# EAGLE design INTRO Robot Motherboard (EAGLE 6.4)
Schematic of the Motherboard from the INTRO Robot
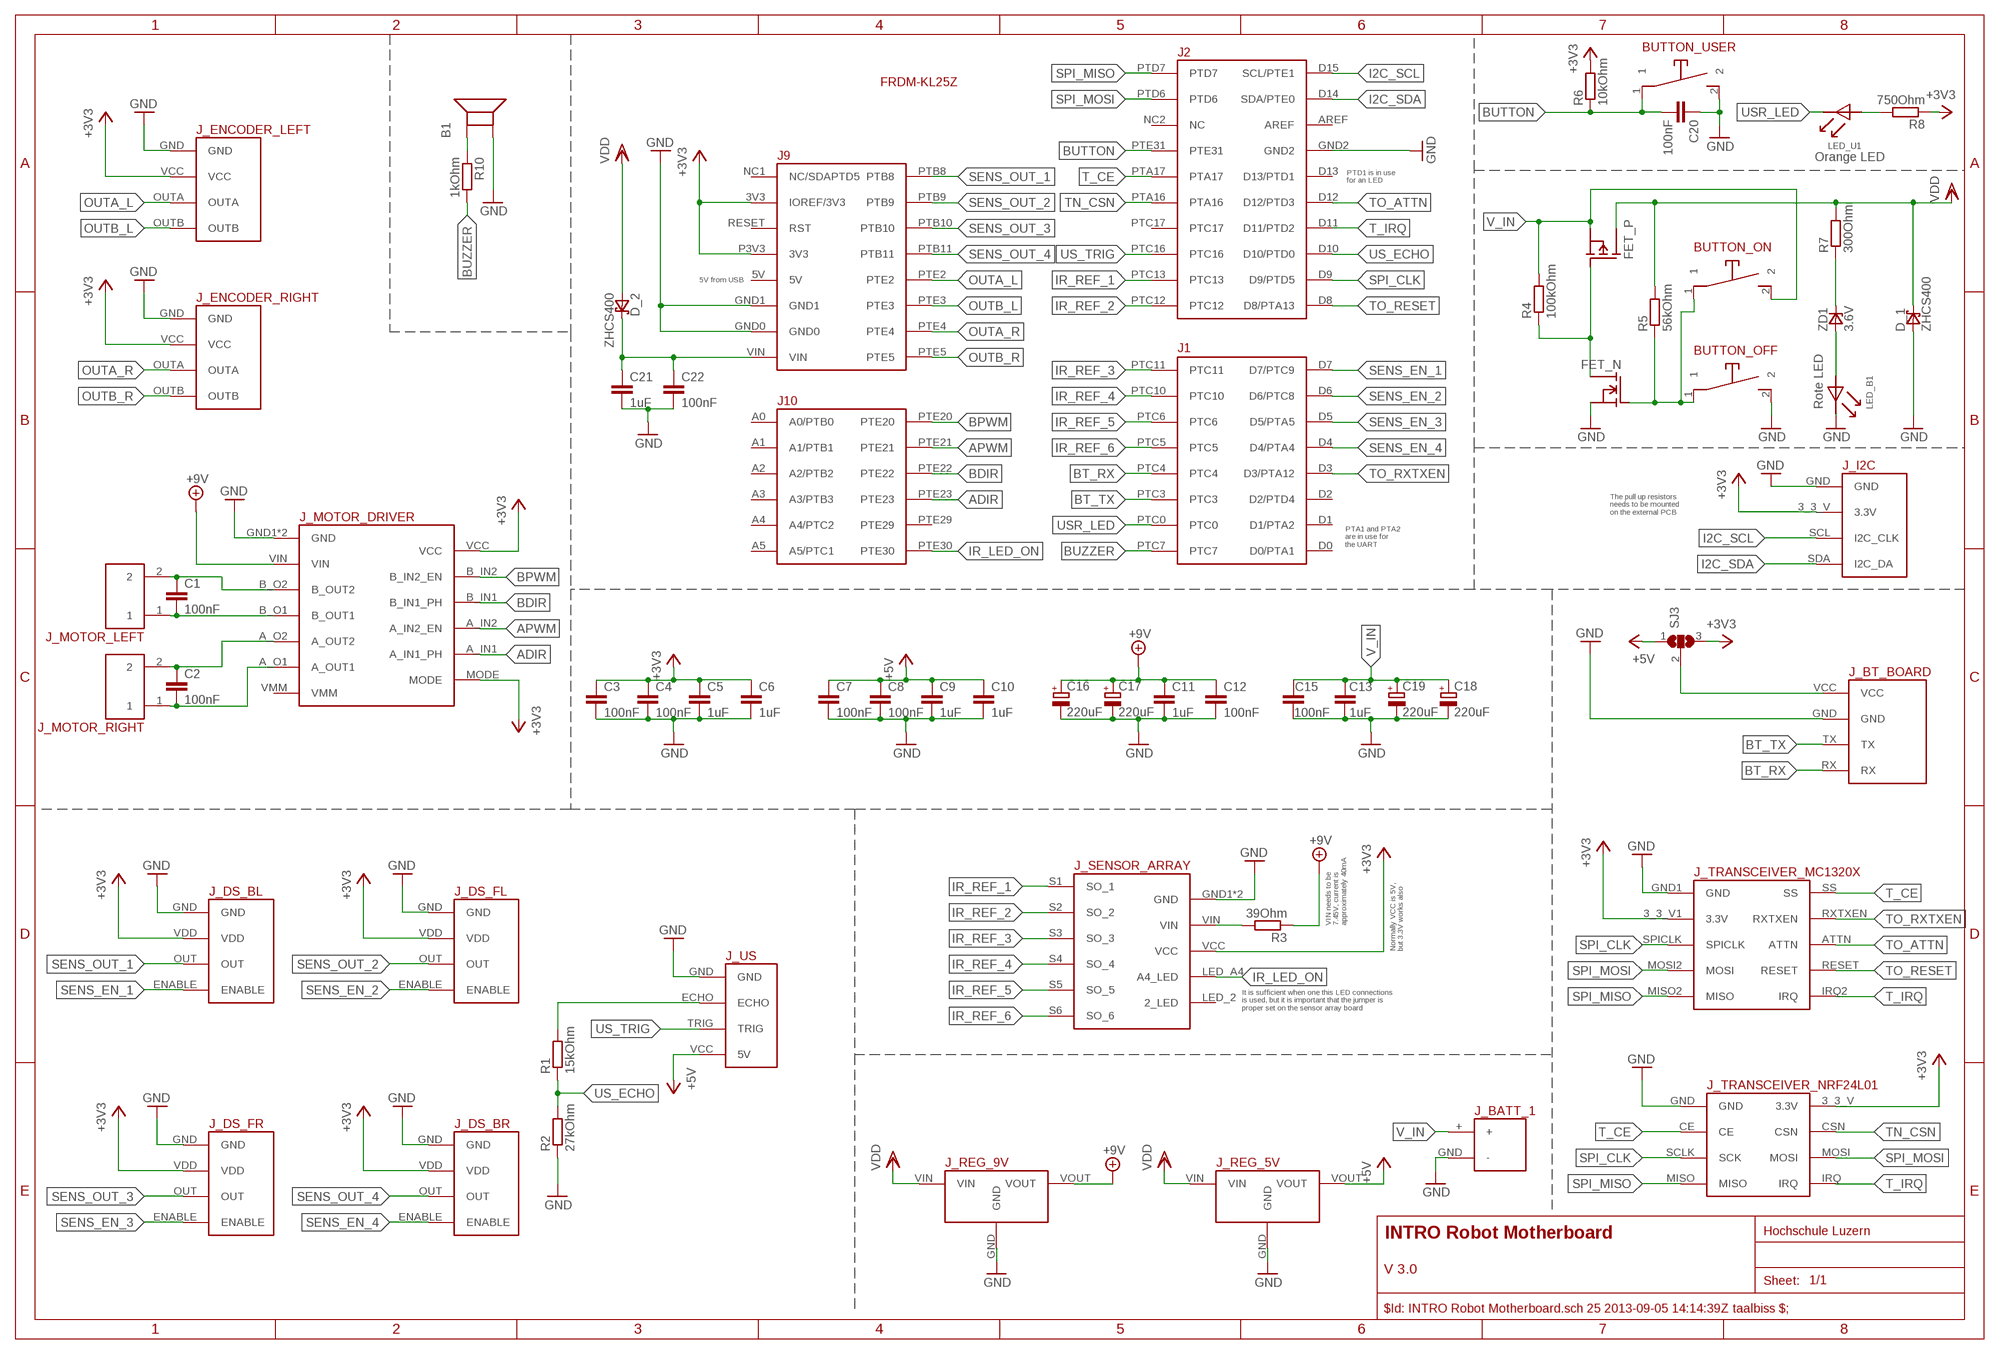
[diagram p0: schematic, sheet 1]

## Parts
B1  BUZZER  [BUZZER]
BUTTON_OFF  MINI_PUSHBUTTON  [MINI_PUSHBUTTON_FOOTPRINT]
BUTTON_ON  MINI_PUSHBUTTON  [MINI_PUSHBUTTON_FOOTPRINT]
BUTTON_USER  MINI_PUSHBUTTON  [MINI_PUSHBUTTON_FOOTPRINT]
C1  100nF  C-EUC0805  [C0805]
C2  100nF  C-EUC0805  [C0805]
C3  100nF  C-EUC0805  [C0805]
C4  100nF  C-EUC0805  [C0805]
C5  1uF  C-EUC0805  [C0805]
C6  1uF  C-EUC0805  [C0805]
C7  100nF  C-EUC0805  [C0805]
C8  100nF  C-EUC0805  [C0805]
C9  1uF  C-EUC0805  [C0805]
C10  1uF  C-EUC0805  [C0805]
C11  1uF  C-EUC0805  [C0805]
C12  100nF  C-EUC0805  [C0805]
C13  1uF  C-EUC0805  [C0805]
C15  100nF  C-EUC0805  [C0805]
C16  220uF  CPOL-EU153CLV-0605  [153CLV-0605]
C17  220uF  CPOL-EU153CLV-0605  [153CLV-0605]
C18  220uF  CPOL-EU153CLV-0605  [153CLV-0605]
C19  220uF  CPOL-EU153CLV-0605  [153CLV-0605]
C20  100nF  C-EUC0805  [C0805]
C21  1uF  C-EUC0805  [C0805]
C22  100nF  C-EUC0805  [C0805]
D_1  ZHCS400  SCHOTTKY_ZHCS400  [SOD-323]
D_2  ZHCS400  SCHOTTKY_ZHCS400  [SOD-323]
FET_N  NFET_SOT23  [SOT-23]
FET_P  PFET_SOT23  [SOT-23]
FRDM1  FRDM-KL25ZARDUINO  [FRDM-KL25Z]
J_BATT_1  BATTERY_CONNECTION  [BATTERY_CONNECTION_FOOTPRINT]
J_BT_BOARD  BLUETOOTH_BOARD  [BT_BOARD_FOOTPRINT]
J_DS_BL  POLOLU_DIST_PROX_SENS  [POLOLU_DIST_PROX_SENS_FOOTPRINT]
J_DS_BR  POLOLU_DIST_PROX_SENS  [POLOLU_DIST_PROX_SENS_FOOTPRINT]
J_DS_FL  POLOLU_DIST_PROX_SENS  [POLOLU_DIST_PROX_SENS_FOOTPRINT]
J_DS_FR  POLOLU_DIST_PROX_SENS  [POLOLU_DIST_PROX_SENS_FOOTPRINT]
J_ENCODER_LEFT  ENCODER  [ENCODER_FOOTPRINT]
J_ENCODER_RIGHT  ENCODER  [ENCODER_FOOTPRINT]
J_I2C  I2C_HEADER  [I2C_HEADER_FOOTPRINT]
J_MOTOR_DRIVER  MOTOR_DRIVER  [MOTOR_DRIVER_FOOTPRINT]
J_MOTOR_LEFT  MOTOR_CONNECTOR  [MOTOR_CONNECTOR_FOOTPRINT]
J_MOTOR_RIGHT  MOTOR_CONNECTOR  [MOTOR_CONNECTOR_FOOTPRINT]
J_REG_5V  5V_VOLTAGE_REGULATOR  [5V_VOLTAGE_REGULATOR]
J_REG_9V  9V_VOLTAGE_REGULATOR  [9V_VOLTAGE_REGULATOR]
J_SENSOR_ARRAY  REFLECTANCE_SENSOR_ARRAY  [REFLECTANCE_SENSOR_ARRAY_FOOTPRINT]
J_TRANSCEIVER  MC1320X_AND_NRF24L01  [MC1320X_AND_NRF24L01_FOOTPRINT]
J_US  HC-SR04  [HC-SR04_FOOTPRINT]
LED_B1  LED_PLCC-2  [PLCC-2]
LED_U1  LED_PLCC-2  [PLCC-2]
R1  15kOhm  R-EU_R0805  [R0805]
R2  27kOhm  R-EU_R0805  [R0805]
R3  39Ohm  R-EU_R0805  [R0805]
R4  100kOhm  R-EU_R0805  [R0805]
R5  56kOhm  R-EU_R0805  [R0805]
R6  10kOhm  R-EU_R0805  [R0805]
R7  300Ohm  R-EU_R0805  [R0805]
R8  750Ohm  R-EU_R0805  [R0805]
R10  1kOhm  R-EU_R0805  [R0805]
SJ3  SJ2W  [SJ_2]
ZD1  3.6V  ZDIODE_SOD323  [SOD-323]

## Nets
+3V3: C3.1 C4.1 C5.1 C6.1 FRDM1.3V3(IOREF/3V3) FRDM1.P3V3(3V3) J_DS_BL.VDD J_DS_BR.VDD J_DS_FL.VDD J_DS_FR.VDD J_ENCODER_LEFT.VCC J_ENCODER_RIGHT.VCC J_I2C.3_3_V(3.3V) J_MOTOR_DRIVER.MODE J_MOTOR_DRIVER.VCC J_SENSOR_ARRAY.VCC J_TRANSCEIVER.3_3_V1(_MC1320X:3.3V) J_TRANSCEIVER.3_3_V(_NRF24L01:3.3V) R6.2 R8.1 SJ3.3
+5V: C7.1 C8.1 C9.1 C10.1 J_REG_5V.VOUT J_US.VCC(5V) SJ3.1
+9V: C11.1 C12.1 C16.+ C17.+ J_MOTOR_DRIVER.VIN J_REG_9V.VOUT R3.1
ADIR: FRDM1.PTE23 J_MOTOR_DRIVER.A_IN1(A_IN1_PH)
APWM: FRDM1.PTE21 J_MOTOR_DRIVER.A_IN2(A_IN2_EN)
BDIR: FRDM1.PTE22 J_MOTOR_DRIVER.B_IN1(B_IN1_PH)
BPWM: FRDM1.PTE20 J_MOTOR_DRIVER.B_IN2(B_IN2_EN)
BT_RX: FRDM1.PTC4 J_BT_BOARD.RX
BT_TX: FRDM1.PTC3 J_BT_BOARD.TX
BUTTON: BUTTON_USER.1 C20.2 FRDM1.PTE31 R6.1
BUZZER: FRDM1.PTC7 R10.2
GND: B1.2 BUTTON_OFF.2 BUTTON_USER.2 C3.2 C4.2 C5.2 C6.2 C7.2 C8.2 C9.2 C10.2 C11.2 C12.2 C13.1 C15.1 C16.- C17.- C18.- C19.- C20.1 C21.2 C22.2 D_1.1(A) FET_N.2(S) FRDM1.GND0 FRDM1.GND1 FRDM1.GND2 J_BATT_1.GND(-) J_BT_BOARD.GND J_DS_BL.GND J_DS_BR.GND J_DS_FL.GND J_DS_FR.GND J_ENCODER_LEFT.GND J_ENCODER_RIGHT.GND J_I2C.GND J_MOTOR_DRIVER.GND1(GND) J_MOTOR_DRIVER.GND2(GND) J_REG_5V.GND J_REG_9V.GND J_SENSOR_ARRAY.GND1(GND) J_SENSOR_ARRAY.GND2(GND) J_TRANSCEIVER.GND1(_MC1320X:GND) J_TRANSCEIVER.GND(_NRF24L01:GND) J_US.GND LED_B1.K R2.1
I2C_SCL: FRDM1.D15(SCL/PTE1) J_I2C.SCL(I2C_CLK)
I2C_SDA: FRDM1.D14(SDA/PTE0) J_I2C.SDA(I2C_DA)
IR_LED_ON: FRDM1.PTE30 J_SENSOR_ARRAY.LED_A4(A4_LED)
IR_REF_1: FRDM1.PTC13 J_SENSOR_ARRAY.S1(SO_1)
IR_REF_2: FRDM1.PTC12 J_SENSOR_ARRAY.S2(SO_2)
IR_REF_3: FRDM1.PTC11 J_SENSOR_ARRAY.S3(SO_3)
IR_REF_4: FRDM1.PTC10 J_SENSOR_ARRAY.S4(SO_4)
IR_REF_5: FRDM1.PTC6 J_SENSOR_ARRAY.S5(SO_5)
IR_REF_6: FRDM1.PTC5 J_SENSOR_ARRAY.S6(SO_6)
N$1: C1.1 J_MOTOR_DRIVER.B_O2(B_OUT2) J_MOTOR_LEFT.2
N$2: J_US.ECHO R1.2
N$3: C2.1 J_MOTOR_DRIVER.A_O2(A_OUT2) J_MOTOR_RIGHT.2
N$4: C1.2 J_MOTOR_DRIVER.B_O1(B_OUT1) J_MOTOR_LEFT.1
N$5: C2.2 J_MOTOR_DRIVER.A_O1(A_OUT1) J_MOTOR_RIGHT.1
N$6: J_SENSOR_ARRAY.VIN R3.2
N$7: C21.1 C22.1 D_2.2(C) FRDM1.VIN
N$8: FET_N.1(D) FET_P.3(G) R4.1
N$9: J_BT_BOARD.VCC SJ3.2
N$10: LED_B1.A ZD1.2(A)
N$11: BUTTON_OFF.1 BUTTON_ON.1 FET_N.3(G) R5.1
N$12: R7.1 ZD1.1(C)
N$15: LED_U1.A R8.2
N$16: B1.1 R10.1
OUTA_L: FRDM1.PTE2 J_ENCODER_LEFT.OUTA
OUTA_R: FRDM1.PTE4 J_ENCODER_RIGHT.OUTA
OUTB_L: FRDM1.PTE3 J_ENCODER_LEFT.OUTB
OUTB_R: FRDM1.PTE5 J_ENCODER_RIGHT.OUTB
SENS_EN_1: FRDM1.D7(D7/PTC9) J_DS_BL.ENABLE
SENS_EN_2: FRDM1.D6(D6/PTC8) J_DS_FL.ENABLE
SENS_EN_3: FRDM1.D5(D5/PTA5) J_DS_FR.ENABLE
SENS_EN_4: FRDM1.D4(D4/PTA4) J_DS_BR.ENABLE
SENS_OUT_1: FRDM1.PTB8 J_DS_BL.OUT
SENS_OUT_2: FRDM1.PTB9 J_DS_FL.OUT
SENS_OUT_3: FRDM1.PTB10 J_DS_FR.OUT
SENS_OUT_4: FRDM1.PTB11 J_DS_BR.OUT
SPI_CLK: FRDM1.D9(D9/PTD5) J_TRANSCEIVER.SCLK(_NRF24L01:SCK) J_TRANSCEIVER.SPICLK(_MC1320X:SPICLK)
SPI_MISO: FRDM1.PTD7 J_TRANSCEIVER.MISO2(_MC1320X:MISO) J_TRANSCEIVER.MISO(_NRF24L01:MISO)
SPI_MOSI: FRDM1.PTD6 J_TRANSCEIVER.MOSI2(_MC1320X:MOSI) J_TRANSCEIVER.MOSI(_NRF24L01:MOSI)
T_CE: FRDM1.PTA17 J_TRANSCEIVER.CE(_NRF24L01:CE) J_TRANSCEIVER.SS(_MC1320X:SS)
T_IRQ: FRDM1.D11(D11/PTD2) J_TRANSCEIVER.IRQ2(_MC1320X:IRQ) J_TRANSCEIVER.IRQ(_NRF24L01:IRQ)
TN_CSN: FRDM1.PTA16 J_TRANSCEIVER.CSN(_NRF24L01:CSN)
TO_ATTN: FRDM1.D12(D12/PTD3) J_TRANSCEIVER.ATTN(_MC1320X:ATTN)
TO_RESET: FRDM1.D8(D8/PTA13) J_TRANSCEIVER.RESET(_MC1320X:RESET)
TO_RXTXEN: FRDM1.D3(D3/PTA12) J_TRANSCEIVER.RXTXEN(_MC1320X:RXTXEN)
US_ECHO: FRDM1.D10(D10/PTD0) R1.1 R2.2
US_TRIG: FRDM1.PTC16 J_US.TRIG
USR_LED: FRDM1.PTC0 LED_U1.K
V_IN: BUTTON_ON.2 C13.2 C15.2 C18.+ C19.+ FET_P.2(S) J_BATT_1.+ R4.2
VDD: D_1.2(C) D_2.1(A) FET_P.1(D) J_REG_5V.VIN J_REG_9V.VIN R5.2 R7.2
Unconnected: FRDM1.5V FRDM1.A0(A0/PTB0) FRDM1.A1(A1/PTB1) FRDM1.A2(A2/PTB2) FRDM1.A3(A3/PTB3) FRDM1.A4(A4/PTC2) FRDM1.A5(A5/PTC1) FRDM1.AREF FRDM1.D0(D0/PTA1) FRDM1.D1(D1/PTA2) FRDM1.D2(D2/PTD4) FRDM1.D13(D13/PTD1) FRDM1.NC1(NC/SDAPTD5) FRDM1.NC2(NC) FRDM1.PTC17 FRDM1.PTE29 FRDM1.RESET(RST) J_MOTOR_DRIVER.VMM J_SENSOR_ARRAY.LED_2(2_LED)

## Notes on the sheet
- Orange LED
- PTD1 is in use
  for an LED
- 5V from USB
- Rote LED
- The pull up resistors 
  needs to be mounted 
  on the external PCB
- PTA1 and PTA2
  are in use for 
  the UART
- VIN needs to be 
  7.45V, current is 
  approximately 40mA
- Normally VCC is 5V, 
  but 3.3V works also
- It is sufficient when one this LED connections 
  is used, but it is important that the jumper is 
  proper set on the sensor array board
- V 3.0
- $Id: INTRO Robot Motherboard.sch 25 2013-09-05 14:14:39Z taalbiss $;

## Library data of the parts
B1 = INTRO_Robot_Miscellaneous:BUZZER
BUTTON_OFF BUTTON_ON BUTTON_USER = Pololu Button:MINI_PUSHBUTTON: Mini Pushbutton Switch, 2-Pin, SPST, 50mA
C1-C13 C15 C20-C22 = rcl:C-EU: CAPACITOR, European symbol
C16-C19 = rcl:CPOL-EU: POLARIZED CAPACITOR, European symbol
D_1 D_2 = INTRO_Robot_Miscellaneous:SCHOTTKY_ZHCS400
FET_N = INTRO_Robot_Miscellaneous:NFET_SOT23
FET_P = INTRO_Robot_Miscellaneous:PFET_SOT23
FRDM1 = Freedom:FRDM-KL25Z: For creating FRDM-KL25Z shields
J_BATT_1 = Zumo Robot Battery Connection:BATTERY_CONNECTION: Battery Connection for the Zuma Robot
J_BT_BOARD = Bluetooth HC-05:BLUETOOTH_BOARD: Bluetooth Board V1.05
J_DS_BL J_DS_BR J_DS_FL J_DS_FR = Pololu Digital Distance and Proximity Sensors:POLOLU_DIST_PROX_SENS: Pololu Digital Distance and Proximity Sensors; Pololu Items Nr. 1134; 1132; 2460; 2461
J_ENCODER_LEFT J_ENCODER_RIGHT = Pololu Encoder and Motor Driver:ENCODER: Encoder for Pololu Wheel 42x19mm
J_I2C = I2C_Header:I2C_HEADER
J_MOTOR_DRIVER = Pololu Encoder and Motor Driver:MOTOR_DRIVER: DRV8835 Dual Motor Driver Carrier
J_MOTOR_LEFT J_MOTOR_RIGHT = Pololu Encoder and Motor Driver:MOTOR_CONNECTOR: Connector for a Motor
J_REG_5V = Pololu Voltage Regulators:5V_VOLTAGE_REGULATOR: Polulu 5V Step-Up/Step-Down Voltage REgulator S7V7F5
J_REG_9V = Pololu Voltage Regulators:9V_VOLTAGE_REGULATOR: Polulu 9V Step-Up Voltage Regulator U3V12F9
J_SENSOR_ARRAY = Pololu Zumo Reflectance Sensor Array:REFLECTANCE_SENSOR_ARRAY: Zumo Reflectance Sensor Array Item #1419
J_TRANSCEIVER = Nordic Semiconductors 2.4GHz Transceiver:MC1320X_AND_NRF24L01: With this Device, it is possible to use the NRF24L01 or the MC1320x 802.15.4 transceiver
J_US = Ultrasonic Sensor HC-SR04:HC-SR04: Ultrasonic Sensor HC-SR04
LED_B1 LED_U1 = INTRO_Robot_Miscellaneous:LED_PLCC-2
R1-R8 R10 = rcl:R-EU_: RESISTOR, European symbol
SJ3 = jumper:SJ2W: SMD solder JUMPER
ZD1 = INTRO_Robot_Miscellaneous:ZDIODE_SOD323

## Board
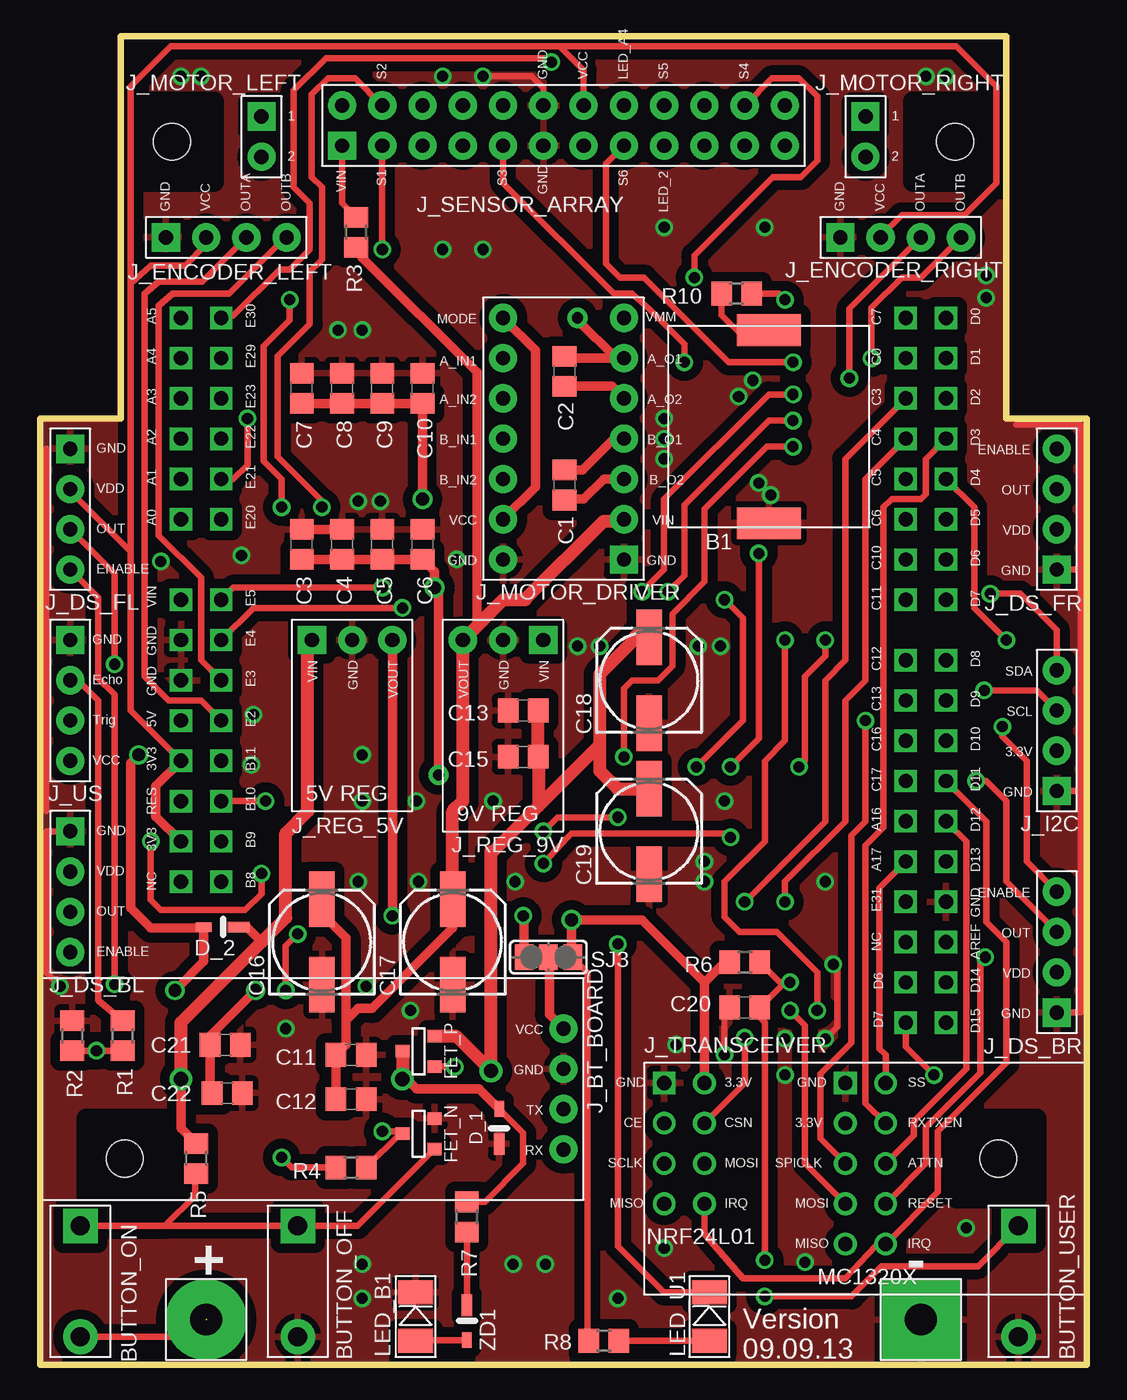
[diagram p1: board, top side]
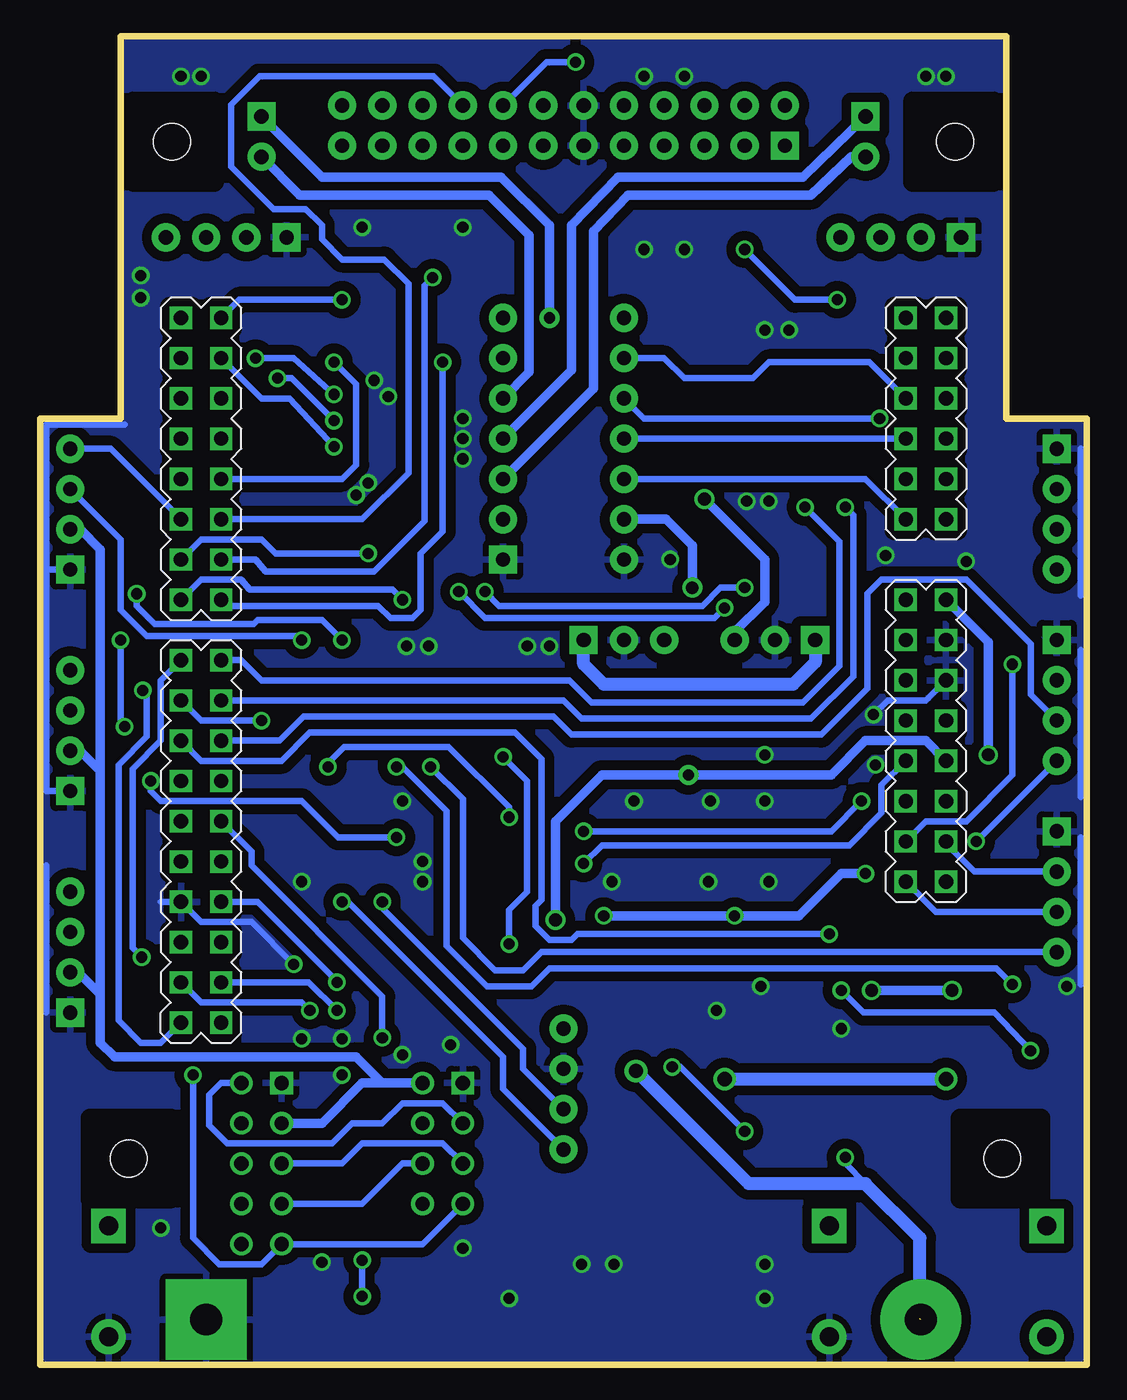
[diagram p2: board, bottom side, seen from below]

No outline drawn. Coordinates in mm, seen from the top.
Copper layers (1*16): 46 0.035mm / dielectric 1.5mm / Bottom 0.035mm
Design rules "default *": minimum track width 10mil, minimum drill 24mil, track to track 10mil, track to pad 10mil, pad to pad 20mil, via to via 20mil, smd to smd 8mil, copper to edge 40mil, drill to drill 10mil, minimum pad ring 10mil, minimum via ring 8mil, stop-mask expansion 4mil, vias tented up to drill 0mil, thermal gap 15mil
Holes 2.31 mm at 5.33,13.02 60.45,13.02 57.72,77.15 8.32,77.15
tRestrict: area 2.9,10.5 to 8,15.6; area 57.8,10.5 to 62.9,15.6; area 5.9,74.6 to 11,79.7; area 55.1,74.6 to 60.1,79.7
bRestrict: area 2.9,10.5 to 8,15.6; area 57.8,10.5 to 62.9,15.6; area 55.1,74.6 to 60.1,79.7; area 5.9,74.6 to 11,79.7
Milling: 8 lines

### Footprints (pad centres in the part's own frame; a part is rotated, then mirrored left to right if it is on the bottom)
BUZZER = smd 2.007 x 4.013: 1 -6.096,0; 2 6.096,0
MINI_PUSHBUTTON_FOOTPRINT = drill 1.2 pad 2.184 square: 1 -3.81,0 | drill 1.2 pad 2.184: 2 3.175,0
C0805 = smd 1.3 x 1.5: 1 -0.95,0; 2 0.95,0
153CLV-0605 = smd 3.5 x 1.6: + 2.7,0; - -2.7,0
SOD-323 = smd 1.397 x 0.66: 1 -1.1,0 | smd 1 x 0.6: 2 1.1,0
SOT-23 = smd 0.787 x 0.889: 1 0.025,-1.016; 2 -0.94,1.016; 3 0.991,1.016
FRDM-KL25Z = drill 0.9 square: 3V3 -22.86,-8.89; 5V -22.86,-1.27; A0 -22.86,11.43; A1 -22.86,13.97; A2 -22.86,16.51; A3 -22.86,19.05; A4 -22.86,21.59; A5 -22.86,24.13; AREF 25.4,-15.24; D0 25.4,24.13; D1 25.4,21.59; D2 25.4,19.05; D3 25.4,16.51; D4 25.4,13.97; D5 25.4,11.43; D6 25.4,8.89; D7 25.4,6.35; D8 25.4,2.54; D9 25.4,0; D10 25.4,-2.54; D11 25.4,-5.08; D12 25.4,-7.62; D13 25.4,-10.16; D14 25.4,-17.78; D15 25.4,-20.32; GND0 -22.86,3.81; GND1 -22.86,1.27; GND2 25.4,-12.7; NC1 -22.86,-11.43; NC2 22.86,-15.24; P3V3 -22.86,-3.81; PTA16 22.86,-7.62; PTA17 22.86,-10.16; PTB8 -20.32,-11.43; PTB9 -20.32,-8.89; PTB10 -20.32,-6.35; PTB11 -20.32,-3.81; PTC0 22.86,21.59; PTC3 22.86,19.05; PTC4 22.86,16.51; PTC5 22.86,13.97; PTC6 22.86,11.43; PTC7 22.86,24.13; PTC10 22.86,8.89; PTC11 22.86,6.35; PTC12 22.86,2.54; PTC13 22.86,0; PTC16 22.86,-2.54; PTC17 22.86,-5.08; PTD6 22.86,-17.78; PTD7 22.86,-20.32; PTE2 -20.32,-1.27; PTE3 -20.32,1.27; PTE4 -20.32,3.81; PTE5 -20.32,6.35; PTE20 -20.32,11.43; PTE21 -20.32,13.97; PTE22 -20.32,16.51; PTE23 -20.32,19.05; PTE29 -20.32,21.59; PTE30 -20.32,24.13; PTE31 22.86,-12.7; RESET -22.86,-6.35; VIN -22.86,6.35
BATTERY_CONNECTION_FOOTPRINT = drill 2 pad 5.08: + -22.86,0 | drill 2 pad 5.08 square: GND 22.225,0
BT_BOARD_FOOTPRINT = drill 0.9 pad 1.778: GND -16.51,-1.27; RX -16.51,3.81; TX -16.51,1.27; VCC -16.51,-3.81
POLOLU_DIST_PROX_SENS_FOOTPRINT = drill 0.9 pad 1.778: ENABLE 0,-3.81; OUT 0,-1.27; VDD 0,1.27 | drill 0.9 pad 1.778 square: GND 0,3.81
ENCODER_FOOTPRINT = drill 0.9 pad 1.778 square: GND -3.81,0 | drill 0.9 pad 1.778: OUTA 1.27,0; OUTB 3.81,0; VCC -1.27,0
I2C_HEADER_FOOTPRINT = drill 0.9 pad 1.778: 3_3_V -1.27,0; SCL 1.27,0; SDA 3.81,0 | drill 0.9 pad 1.778 square: GND -3.81,0
MOTOR_DRIVER_FOOTPRINT = drill 0.9 pad 1.778: A_IN1 3.81,-5.08; A_IN2 3.81,-2.54; A_O1 -3.81,-5.08; A_O2 -3.81,-2.54; B_IN1 3.81,0; B_IN2 3.81,2.54; B_O1 -3.81,0; B_O2 -3.81,2.54; GND2 3.81,7.62; MODE 3.81,-7.62; VCC 3.81,5.08; VIN -3.81,5.08; VMM -3.81,-7.62 | drill 0.9 pad 1.778 square: GND1 -3.81,7.62
MOTOR_CONNECTOR_FOOTPRINT = drill 0.9 pad 1.778 square: 1 0,1.27 | drill 0.9 pad 1.778: 2 0,-1.27
5V_VOLTAGE_REGULATOR = drill 0.9 pad 1.778: GND 0,-6.35; VOUT -2.54,-6.35 | drill 0.9 pad 1.778 square: VIN 2.54,-6.35
9V_VOLTAGE_REGULATOR = drill 0.9 pad 1.778: GND 0,-1.27; VOUT 2.54,-1.27 | drill 0.9 pad 1.778 square: VIN -2.54,-1.27
REFLECTANCE_SENSOR_ARRAY_FOOTPRINT = drill 0.9 pad 1.778: GND1 -1.27,0; GND2 1.27,0; LED_2 -1.27,-7.62; LED_A4 1.27,-5.08; NC$4 1.27,2.54; NC$5 -1.27,5.08; NC$6 1.27,5.08; NC$7 -1.27,7.62; NC$8 1.27,7.62; NC$12 1.27,12.7; NC$15 -1.27,-2.54; NC$17 -1.27,-10.16; NC$18 1.27,-10.16; NC$21 -1.27,-12.7; NC$23 -1.27,-15.24; NC$24 1.27,-15.24; S1 -1.27,10.16; S2 1.27,10.16; S3 -1.27,2.54; S4 1.27,-12.7; S5 1.27,-7.62; S6 -1.27,-5.08; VCC 1.27,-2.54 | drill 0.9 pad 1.778 square: VIN -1.27,12.7
MC1320X_AND_NRF24L01_FOOTPRINT = drill 0.9 pad 1.422: 3_3_V -11.43,6.35; 3_3_V1 -2.54,3.81; ATTN 0,1.27; CE -13.97,3.81; CSN -11.43,3.81; IRQ -11.43,-1.27; IRQ2 0,-3.81; MISO -13.97,-1.27; MISO2 -2.54,-3.81; MOSI -11.43,1.27; MOSI2 -2.54,-1.27; RESET 0,-1.27; RXTXEN 0,3.81; SCLK -13.97,1.27; SPICLK -2.54,1.27; SS 0,6.35 | drill 0.9 pad 1.422 square: GND -13.97,6.35; GND1 -2.54,6.35
HC-SR04_FOOTPRINT = drill 0.9 pad 1.778: ECHO 0,1.27; TRIG 0,-1.27; VCC 0,-3.81 | drill 0.9 pad 1.778 square: GND 0,3.81
PLCC-2 = smd 1.499 x 2.21: A -1.524,0; K 1.524,0
R0805 = smd 1.3 x 1.5: 1 -0.95,0; 2 0.95,0
SJ_2 = smd 1.168 x 1.6: 1 -1.524,0; 2 0,0; 3 1.524,0

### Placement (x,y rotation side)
B1  45.97,59.18 270 top
BUTTON_OFF  16.26,4.95 270 top
BUTTON_ON  2.54,4.95 270 top
BUTTON_USER  61.72,4.95 270 top
C1  33.08,55.5 90 top
C2  33.08,62.67 90 top
C3  16.51,51.75 90 top
C4  19.05,51.75 90 top
C5  21.59,51.75 90 top
C6  24.13,51.75 90 top
C7  16.51,61.59 90 top
C8  19.05,61.59 90 top
C9  21.59,61.59 90 top
C10  24.13,61.59 90 top
C11  19.62,19.56 0 top
C12  19.62,16.76 0 top
C13  30.48,41.27 0 top
C15  30.48,38.35 0 top
C16  17.78,26.67 90 top
C17  26.04,26.67 90 top
C18  38.42,43.18 90 top
C19  38.42,33.66 90 top
C20  44.45,22.54 0 top
C21  11.68,20.19 0 top
C22  11.81,17.14 0 top
D_1  28.96,15.05 90 top
D_2  11.43,27.62 180 top
FET_N  23.88,14.61 270 top
FET_P  23.88,19.81 270 top
FRDM1  31.75,41.91 0 top
J_BATT_1  33.34,2.86 0 top
J_BT_BOARD  16.51,17.4 180 top
J_DS_BL  1.91,29.84 0 top
J_DS_BR  64.14,26.04 180 top
J_DS_FL  1.91,53.98 0 top
J_DS_FR  64.14,53.98 180 top
J_ENCODER_LEFT  11.75,71.12 0 top
J_ENCODER_RIGHT  54.29,71.12 0 top
J_I2C  64.14,40.01 90 top
J_MOTOR_DRIVER  33.02,58.42 180 top
J_MOTOR_LEFT  13.97,77.47 0 top
J_MOTOR_RIGHT  52.07,77.47 0 top
J_REG_5V  19.68,39.37 180 top
J_REG_9V  29.21,44.45 180 top
J_SENSOR_ARRAY  31.75,78.17 90 top
J_TRANSCEIVER  53.34,11.43 0 top
J_US  1.91,41.91 0 top
LED_B1  23.69,3.05 90 top
LED_U1  42.23,3.05 90 top
R1  5.21,20.76 90 top
R2  2.03,20.76 270 top
R3  19.94,71.44 90 top
R4  19.62,12.45 180 top
R5  9.84,13.02 90 top
R6  44.45,25.4 180 top
R7  26.92,9.33 90 top
R8  35.56,1.52 0 top
R10  43.94,67.56 0 top
SJ3  32.07,25.72 0 top
ZD1  26.92,2.67 270 top

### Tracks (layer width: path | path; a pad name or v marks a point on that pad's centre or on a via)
+3V3  (via drill 0.7 pad 1.27, 0.8 pad 1.27)
  46 0.406: 5.71,68.2 5.71,51.31 | 5.71,51.31 5.71,41.27 FRDM1.P3V3 | J_ENCODER_LEFT.VCC 10.48,70.67 9.14,69.34 6.99,69.34 5.71,68.2 | SJ3.3 34.54,24.77 34.54,1.59 R8.1 | 32.77,83.19 8.26,83.19 5.71,80.64 5.71,68.2 | 32.77,83.19 57.78,83.19 60.33,80.64 60.33,74.55 58.29,72.52 54.36,72.52 53.02,71.18 J_ENCODER_RIGHT.VCC | J_DS_FL.VDD 1.91,55.12 5.71,51.31 | J_SENSOR_ARRAY.VCC 34.29,81.66 32.77,83.19
  46 0.61: C3.1 | FRDM1.P3V3 7.3,36.51 7.3,34.61 FRDM1.3V3 | 33.91,25.4 SJ3.3 33.53,25.78 v33.53,28.07 37.97,28.07 41.91,24.13 | R6.2 43.18,25.4 41.91,24.13 | C3.1 C4.1 | C3.1 C5.1 C6.1 | C3.1 23.75,50.8 | J_MOTOR_DRIVER.MODE 31.24,64.01 31.24,55.37 J_MOTOR_DRIVER.VCC | 41.91,24.13 J_TRANSCEIVER.3_3_V | C6.1 | v25.15,37.21 25.15,48.77 v24.89,49.02 24.89,50.04 C6.1
  Bottom 0.406: FRDM1.3V3 8.89,32.89 7.11,31.11 J_DS_BL.VDD
  Bottom 0.61: 62.23,37.47 62.23,51.44 63.5,52.7 J_DS_FR.VDD | 62.23,37.47 62.23,23.37 | 62.23,23.37 62.23,20.32 61.34,19.43 46.1,19.43 44.45,17.78 | 44.45,17.78 45.72,17.78 48.26,15.24 J_TRANSCEIVER.3_3_V1 | 44.45,17.78 J_TRANSCEIVER.3_3_V | FRDM1.P3V3 10.16,39.37 13.97,39.37 16.13,37.21 v25.15,37.21 30.61,37.21 33.53,34.29 v33.53,28.07 | J_I2C.3_3_V 63.5,38.73 62.23,37.47 | J_DS_BR.VDD 63.63,24.77 62.23,23.37 | v24.89,49.02 24.89,51.69 26.54,53.34 J_MOTOR_DRIVER.VCC
+5V  (via drill 0.7, 0.8 pad 1.27)
  46 0.406: v6.99,33.02 6.99,29.34 7.62,28.7 12.95,28.7 13.97,29.72 v13.97,30.99
  46 0.61: C10.1 C9.1 | C10.1 C8.1 C7.1 | SJ3.1 30.54,28.26 v30.48,28.32 | J_REG_5V.VOUT v22.23,28.32 | v24.13,54.61 C10.1
  Bottom 0.406: J_US.VCC v6.99,33.02
  Bottom 0.61: J_REG_5V.VOUT 22.23,46.23 20.32,48.13 20.32,50.8 v24.13,54.61 | v13.97,30.99 15.49,30.99 18.16,28.32 v22.23,28.32 v30.48,28.32
+9V
  46 0.61: C12.1 C11.1 19.3,20.19 19.3,21.72 | 26.04,28.57 C17.+ 26.04,27.56 20.95,22.48 20.07,22.48 19.3,21.72 | C16.+ 17.78,28.45 19.3,26.92 19.3,21.72 | J_REG_9V.VOUT 27.56,46.61 27.56,62.61 20.32,69.85 20.32,70.11 R3.1
  46 0.813: 36.7,53.21 35.56,53.21 30.61,48.26 29.21,48.26 J_REG_9V.VOUT 26.67,35.56 26.04,34.92 C17.+
  46 1.016: 36.7,53.21 J_MOTOR_DRIVER.VIN
ADIR
  Bottom 0.406: FRDM1.PTE23 13.72,63.25 20.07,63.25 21.08,62.23 25.4,62.23 26.67,63.5 J_MOTOR_DRIVER.A_IN1
APWM  (via drill 0.7)
  46 0.406: FRDM1.PTE21 12.19,55.88 13.08,56.77 v13.08,59.69
  Bottom 0.406: v13.08,59.69 27.94,59.69 J_MOTOR_DRIVER.A_IN2
BDIR
  Bottom 0.406: FRDM1.PTE22 J_MOTOR_DRIVER.B_IN1
BPWM
  Bottom 0.406: J_MOTOR_DRIVER.B_IN2 13.97,55.88 FRDM1.PTE20
BT_RX  (via drill 0.7 pad 1.02)
  46 0.406: FRDM1.PTC4 52.07,55.88 52.07,43.18 50.8,41.91 50.8,34.29 46.99,30.48 v46.99,29.21
  Bottom 0.406: v46.99,29.21 46.61,29.21 36.83,19.43 36.83,17.4 J_BT_BOARD.RX
BT_TX  (via drill 0.7 pad 1.02)
  46 0.406: FRDM1.PTC3 50.8,57.15 50.8,44.45 49.53,43.18 49.53,34.29 v44.45,29.21
  Bottom 0.406: v44.45,29.21 44.45,28.83 35.56,19.94 35.56,18.67 J_BT_BOARD.TX
BUTTON  (via drill 0.7, 0.7 pad 1.02)
  46 0.406: 46.99,24.13 46.67,24.13 R6.1 | 46.99,24.13 C20.2 45.4,21.91 45.72,21.59 v45.72,6.6 | 46.99,24.13 v47.3,24.13 | v45.72,4.32 51.18,4.32 53.09,6.22 59.18,6.22 BUTTON_USER.1
  Bottom 0.406: v45.72,4.32 v45.72,6.6 | 53.34,29.21 FRDM1.PTE31 52.32,29.21 47.3,24.19 v47.3,24.13
BUZZER  (via drill 0.7 pad 1.02)
  46 0.406: R10.2 46.61,67.56 v46.99,67.18
  Bottom 0.406: v46.99,67.18 53.47,67.18 FRDM1.PTC7
GND  (via drill 0.7, 0.7 pad 1.02)
  46 0.406: v43.18,19.56 43.18,22.22 C20.1 | J_SENSOR_ARRAY.GND2 31.75,80.52 30.99,81.28 v27.94,81.28 | J_DS_BR.GND 65.66,22.23 65.66,36.2 | J_I2C.GND 65.66,36.2 | 65.66,36.2 65.66,50.16 | 65.66,50.16 J_DS_FR.GND | J_DS_BL.GND 0.38,33.66 0.38,24.77 v1.27,23.88 | v50.04,25.27 50.29,25.02 50.29,21.34 v49.53,20.57 | 0.38,57.78 0.38,34.92 | 65.66,50.16 65.66,59.31 61.59,59.31
  46 0.61: C4.2 C3.2
  Bottom 0.406: J_I2C.GND 65.66,36.2 65.66,50.04 | 65.66,50.04 65.53,50.16 J_DS_FR.GND | 65.66,50.04 65.66,59.31 60.71,59.31 | 65.66,22.23 65.66,31.5 | 0.38,24 0.38,33.27 | 0.38,35.81 0.38,45.09 | FRDM1.GND1 10.16,41.91 12.57,41.91 v13.46,41.02 | 58.42,29.21 FRDM1.GND2 55.88,27.94 52.7,27.94 v50.04,25.27 | 0.38,48.51 0.38,57.78
  other vias: 46.99,18.29 39.37,59.69 39.37,57.15 39.37,58.42 44.96,62.1 44.07,61.09 45.34,55.63 46.1,54.86 41.91,31.75 41.91,30.48 57.15,81.28 55.88,81.28 8.89,81.28 10.16,81.28 41.53,45.34 42.93,45.34 35.31,45.34 33.91,45.34 20.07,54.48 21.46,54.48 20.32,38.48 20.32,35.56 28.57,35.56 20.07,30.48 29.97,30.48 20.57,23.88 23.37,22.35 15.49,21.21 18.8,65.28 20.32,65.28 25.4,70.36 27.94,70.36 25.4,81.28 7.62,50.67 12.7,51.05 13.34,37.85 59.69,68.71 59.69,67.31 29.84,6.35 31.88,6.35 20.32,6.35 20.32,4.19 36.45,4.19 26.29,50.8 23.75,35.56 43.18,35.56 46.99,20.57 49.53,30.48 48.26,6.48 40.13,20.19 39.37,7.37 45.72,71.75 39.37,71.75 23.88,30.48 58.42,8.64
  pour Bottom (isolate 0.61): 0.38,0.38 0.38,59.31 5.46,59.31 5.46,83.44 60.58,83.44 60.58,59.31 65.66,59.31 65.66,0.38
  pour 46 (isolate 0.61): 0.38,0.38 0.38,59.31 5.46,59.31 5.46,64.14 5.46,83.44 60.58,83.44 60.58,72.64 60.58,59.31 65.66,59.31 65.66,59.05 65.66,41.66 65.66,27.81 65.66,14.73 65.66,2.92 65.66,0.38
I2C_SCL  (via drill 0.7 pad 1.02)
  46 0.406: v59.56,42.55 62.87,42.55 J_I2C.SCL
  Bottom 0.406: FRDM1.D15 58.42,20.32 59.69,20.32 61.09,21.72 61.09,37.85 59.31,39.62 59.31,42.29 v59.56,42.55
I2C_SDA  (via drill 0.7, 0.7 pad 1.02)
  46 0.406: v46.99,45.72 46.99,39.37 45.72,38.1 45.72,33.02 43.18,30.48 43.18,28.26 44.13,27.3 46.48,27.3 49.02,24.77 v49.02,22.35 | v59.94,48.64 61.85,48.64 64.14,46.35 J_I2C.SDA
  Bottom 0.406: FRDM1.D14 55.88,22.86 49.53,22.86 v49.02,22.35 | v46.99,45.72 48.26,46.99 52.32,46.99 52.58,46.74 58.8,46.74 59.94,47.88 v59.94,48.64
IR_LED_ON  (via drill 0.7)
  46 0.406: FRDM1.PTE30 11.56,66.17 12.19,66.17 15.11,69.09 15.75,69.09 17.02,70.36 17.02,73.28 16,74.3 16,80.39 18.03,82.42 32,82.42 v32.26,82.17
  Bottom 0.406: J_SENSOR_ARRAY.LED_A4 34.1,82.17 v32.26,82.17
IR_REF_1  (via drill 0.7, 0.7 pad 1.02)
  46 0.406: v15.24,54.1 15.24,55.88 14.1,57.02 14.1,64.26 15.75,65.91 v15.75,67.18 | v21.59,70.36 J_SENSOR_ARRAY.S1
  Bottom 0.406: FRDM1.PTC13 33.02,41.91 31.88,40.77 19.94,40.77 19.43,40.77 17.4,40.77 14.73,43.43 14.73,53.59 v15.24,54.1 | v15.75,67.18 18.41,67.18 v21.59,70.36
IR_REF_2  (via drill 0.7 pad 1.02)
  46 0.406: v17.78,54.1 17.78,54.48 14.99,57.28 14.99,63.63 17.02,65.66 17.02,68.96 17.78,69.72 17.78,74.3 17.14,74.93 17.14,80.14 18.16,81.15 19.88,81.15 J_SENSOR_ARRAY.S2
  Bottom 0.406: FRDM1.PTC12 53.34,44.45 52.07,43.18 32.64,43.18 31.24,41.78 20.45,41.78 19.94,41.78 17.91,41.78 15.62,44.07 15.62,51.94 v17.78,54.1
IR_REF_3  (via drill 0.7 pad 1.02)
  46 0.406: v40.64,63.25 40.64,64.39 38.48,66.55 37.34,67.56 36.2,67.56 29.21,74.55 J_SENSOR_ARRAY.S3
  Bottom 0.406: FRDM1.PTC11 54.36,47.88 44.7,47.88 43.94,47.12 42.55,47.12 42.04,47.62 42.04,51.18 40.64,52.58 v40.64,63.25
IR_REF_4  (via drill 0.7 pad 1.02)
  46 0.406: J_SENSOR_ARRAY.S4 46.16,81.15 47.88,81.15 49.02,80.01 49.02,75.95 48.01,74.93 46.23,74.93 41.27,69.98 v41.27,68.58
  Bottom 0.406: FRDM1.PTC10 52.45,50.8 51.82,50.04 44.96,50.04 41.78,53.21 41.78,68.07 v41.27,68.58 41.53,68.33
IR_REF_5
  Bottom 0.406: FRDM1.PTC6 45.72,53.34 42.8,56.26 42.8,68.2 44.32,69.72 46.99,69.72 48.26,70.99 48.26,71.88 49.28,72.9 51.31,72.9 53.98,75.56 53.98,79.5 52.2,81.28 41.21,81.28 J_SENSOR_ARRAY.S5
IR_REF_6  (via drill 0.7 pad 1.02)
  46 0.406: v47.5,63.25 43.43,63.25 38.1,68.58 36.58,68.58 35.69,69.47 35.69,75.75 J_SENSOR_ARRAY.S6
  Bottom 0.406: FRDM1.PTC5 46.99,55.88 46.1,56.77 46.1,61.85 v47.5,63.25
N$1
  46 0.61: C1.1 33.15,54.61 34.29,54.61 35.56,55.88 J_MOTOR_DRIVER.B_O2
  Bottom 0.61: J_MOTOR_DRIVER.B_O2 31.11,61.59 31.11,71.5 28.96,73.79 17.4,73.79 14.86,76.2 J_MOTOR_LEFT.2
N$2
  46 0.406: J_US.ECHO 2.41,43.18 3.68,41.91 3.68,22.98 R1.2
N$3
  46 0.61: C2.1 36.07,61.72 J_MOTOR_DRIVER.A_O2
  Bottom 0.61: J_MOTOR_DRIVER.A_O2 35.18,62.61 35.18,71.25 37.72,73.79 49.66,73.79 J_MOTOR_RIGHT.2
N$4
  46 0.61: C1.2 34.22,56.45 36.2,58.42 J_MOTOR_DRIVER.B_O1
  Bottom 0.61: J_MOTOR_LEFT.1 17.91,74.93 29.59,74.93 32.51,71.88 32.51,62.74 J_MOTOR_DRIVER.B_O1
N$5  (via drill 0.7 pad 1.27)
  46 0.61: J_MOTOR_DRIVER.A_O1 36.32,63.5 | 36.32,63.5 33.21,63.5 C2.2 | v33.91,66.04 33.91,65.91 36.32,63.5
  Bottom 0.61: v33.91,66.04 33.91,71.88 36.96,74.93 48.26,74.93 J_MOTOR_RIGHT.1
N$6
  46 0.406: J_SENSOR_ARRAY.VIN 19.05,73.28 R3.2
N$7  (via drill 0.8)
  46 0.61: v8.51,23.62 10.33,25.44 D_2.2 10.27,27.56 6.99,27.56 5.71,28.83 5.71,37.97 v6.22,38.48 | v13.59,23.62 10.79,20.83 10.79,20.25 C21.1 10.73,17.27 C22.1
  Bottom 0.61: v6.22,38.48 6.22,45.59 FRDM1.VIN | v8.51,23.62 v13.59,23.62
N$8  (via drill 0.7)
  46 0.406: 20.65,12.45 R4.1 22.7,14.58 FET_N.1 22.71,14.73 v21.59,14.73 | FET_P.3 26.14,18.82 v26.16,18.8
  Bottom 0.406: v26.16,18.8 25.65,18.8 v21.59,14.73
N$9
  46 0.61: SJ3.2 32.13,25.72 32.13,22.1 J_BT_BOARD.VCC
N$10
  46 0.406: ZD1.2 23.73,1.57 LED_B1.A
N$11
  46 0.406: BUTTON_ON.1 7.87,8.76 | 7.87,8.76 9.78,10.67 9.78,12 R5.1 | 7.87,8.76 BUTTON_OFF.1 20.04,8.76 FET_N.3
N$12
  46 0.406: ZD1.1 R7.1
N$15
  46 0.406: R8.2 LED_U1.A
N$16
  46 0.406: R10.1 42.99,66.23 44.45,64.77 45.47,64.77 B1.1
OUTA_L
  46 0.406: FRDM1.PTE2 10.16,41.91 8.13,41.91 6.6,43.43 6.6,67.56 7.49,68.33 10.22,68.33 J_ENCODER_LEFT.OUTA
OUTA_R  (via drill 0.7 pad 1.02)
  46 0.406: 55.37,71.12 J_ENCODER_RIGHT.OUTA 51.05,66.61 v51.05,62.23 | v22.86,47.75 13.46,47.75 FRDM1.PTE4 | v39.62,48.77 40.64,49.78 40.64,54.23 45.97,59.56 v47.5,59.56
  Bottom 0.406: v47.5,59.56 50.16,62.23 v51.05,62.23 | v22.86,47.75 23.5,47.12 37.97,47.12 v39.62,48.77
OUTB_L
  46 0.406: J_ENCODER_LEFT.OUTB 15.49,71.12 11.94,67.56 8.38,67.56 7.49,66.8 7.49,52.32 10.16,49.66 10.16,44.45 FRDM1.PTE3
OUTB_R  (via drill 0.7 pad 1.02)
  46 0.406: J_ENCODER_RIGHT.OUTB 55.56,68.58 54.36,68.58 52.45,66.67 v52.45,63.5 | v37.97,48.77 39.37,50.16 39.37,54.61 45.97,61.21 v47.5,61.21 | v21.59,49.02 12.19,49.02 FRDM1.PTE5
  Bottom 0.406: v47.5,61.21 50.04,63.5 v52.45,63.5 | v37.97,48.77 37.08,47.88 24.26,47.88 23.11,49.02 v21.59,49.02
SENS_EN_1  (via drill 0.7 pad 1.02)
  46 0.406: v43.18,48.26 44.32,47.12 44.32,40.64 v41.4,37.72
  Bottom 0.406: FRDM1.D7 55.88,49.53 53.34,49.53 52.83,48.9 43.81,48.9 v43.18,48.26 | J_DS_BL.ENABLE 34.42,26.04 35.56,24.89 37.34,24.89 39.37,26.92 39.37,35.69 v41.4,37.72
SENS_EN_2  (via drill 0.7 pad 1.02)
  46 0.406: v45.34,51.18 45.34,39.5 v43.56,37.72 | J_DS_FL.ENABLE 3.68,48.39 3.68,43.31 4.7,42.29 v4.7,24
  Bottom 0.406: FRDM1.D6 55.88,52.07 52.07,52.07 51.18,51.18 v45.34,51.18 | v4.7,24 5.71,25.02 33.91,25.02 35.05,23.88 37.85,23.88 40.39,26.42 40.39,34.92 43.18,37.72 v43.56,37.72
SENS_EN_3
  Bottom 0.406: FRDM1.D5 61.59,57.78 J_DS_FR.ENABLE
SENS_EN_4  (via drill 0.7)
  46 0.406: J_DS_BR.ENABLE 62.23,31.75 62.23,38.1 60.71,39.62 v60.71,40.26 | v60.96,45.72 58.93,47.75 58.93,54.1 FRDM1.D4
  Bottom 0.406: v60.96,45.72 60.96,40.51 v60.71,40.26
SENS_OUT_1
  Bottom 0.406: FRDM1.PTB8 9.53,28.57 J_DS_BL.OUT
SENS_OUT_2  (via drill 0.7)
  46 0.406: J_DS_FL.OUT 4.7,49.91 v4.7,44.2
  Bottom 0.406: FRDM1.PTB9 10.16,34.29 7.62,34.29 4.7,37.21 v4.7,44.2
SENS_OUT_3  (via drill 0.7, 0.7 pad 1.02)
  46 0.406: v49.53,45.72 49.53,44.7 48.26,43.43 48.26,38.1 v47.88,37.72 | v14.22,35.56 FRDM1.PTB10 | v36.45,34.54 32.64,34.54 v31.75,33.66
  Bottom 0.406: v31.75,33.66 16.13,33.66 v14.22,35.56 | J_DS_FR.OUT 60.96,52.07 60.96,47.62 59.31,45.97 49.78,45.97 v49.53,45.72 | v47.88,37.72 47.88,37.97 46.86,38.99 40.26,38.99 36.45,35.18 v36.45,34.54
SENS_OUT_4  (via drill 0.7 pad 1.02)
  46 0.406: v59.05,36.83 59.69,36.83 60.96,35.56 60.96,30.48 J_DS_BR.OUT | v31.75,31.62 33.27,33.27 33.53,33.53 43.31,33.53 v43.56,33.27
  Bottom 0.406: v43.56,33.27 47.24,33.27 49.53,35.56 58.42,35.56 59.05,36.2 v59.05,36.83 | FRDM1.PTB11 12.95,36.58 12.95,34.8 14.99,32.77 30.61,32.77 v31.75,31.62
SPI_CLK  (via drill 0.7 pad 1.02)
  46 0.406: J_TRANSCEIVER.SPICLK 49.21,14.29 49.21,18.35 51.18,20.32 51.18,33.4 52.07,34.29 v52.07,40.64
  Bottom 0.406: J_TRANSCEIVER.SCLK 40.64,13.97 45.72,13.97 46.99,12.7 J_TRANSCEIVER.SPICLK | v52.07,40.64 55.88,40.64 FRDM1.D9
SPI_MISO  (via drill 0.7 pad 1.02)
  46 0.406: FRDM1.PTD7 54.61,20.07 v56.39,18.29
  Bottom 0.406: J_TRANSCEIVER.MISO 41.91,7.62 J_TRANSCEIVER.MISO2 52.07,6.35 54.74,6.35 56.39,8 v56.39,18.29
SPI_MOSI  (via drill 0.7 pad 1.02)
  46 0.406: J_TRANSCEIVER.MOSI2 48.26,12.7 48.26,21.4 v47.31,22.35
  Bottom 0.406: J_TRANSCEIVER.MOSI2 45.72,10.16 43.18,12.7 J_TRANSCEIVER.MOSI | FRDM1.PTD6 49.09,24.13 v47.31,22.35
T_CE
  46 0.406: J_TRANSCEIVER.SS 53.34,19.56 52.96,19.94 52.96,30.1 FRDM1.PTA17
  Bottom 0.406: J_TRANSCEIVER.CE 40.64,16.51 43.18,16.51 44.45,15.24 46.35,15.24 47.62,13.97 54.23,13.97 55.37,15.11 55.37,17.02 54.61,17.78 J_TRANSCEIVER.SS
T_IRQ
  46 0.406: J_TRANSCEIVER.IRQ 41.91,8.26 44.32,5.46 50.8,5.46 52.7,7.49 53.21,7.49 J_TRANSCEIVER.IRQ2 56.64,10.92 56.64,14.73 60.96,19.05 60.96,26.67 59.69,27.94 59.69,34.29 FRDM1.D11
TN_CSN  (via drill 0.7 pad 1.02)
  46 0.406: J_TRANSCEIVER.CSN 44.45,17.78 v44.45,20.64
  Bottom 0.406: v44.45,20.64 44.45,23.24 52.7,31.5 52.7,32.38 FRDM1.PTA16
TO_ATTN
  46 0.406: FRDM1.D12 58.42,33.02 58.42,18.67 55.12,15.37 55.12,14.48 J_TRANSCEIVER.ATTN
TO_RESET  (via drill 0.7 pad 1.02)
  46 0.406: J_TRANSCEIVER.RESET 55.88,12.7 55.88,14.99 59.31,18.41 59.31,25.4 v59.63,25.72
  Bottom 0.406: FRDM1.D8 58.42,43.18 58.42,39.37 60.2,37.59 60.2,26.29 v59.63,25.72
TO_RXTXEN
  46 0.406: FRDM1.D3 55.88,57.15 55.88,54.93 55.56,54.61 53.72,54.61 53.21,54.1 53.21,33.91 52.07,32.77 52.07,16.51 J_TRANSCEIVER.RXTXEN
US_ECHO  (via drill 0.7)
  46 0.406: R1.1 4.95,19.81 v3.56,19.81 3.43,19.81 R2.2 | v15.49,23.62 15.49,26.42 v16.26,27.18
  Bottom 0.406: FRDM1.D10 55.88,38.1 50.8,38.1 49.02,39.88 36.07,39.88 34.42,38.23 34.42,29.34 34.8,28.96 34.8,27.69 33.91,26.8 32.51,26.8 32.13,27.18 v16.26,27.18 | v3.56,19.81 5.84,22.23 14.1,22.23 v15.49,23.62
US_TRIG
  Bottom 0.406: J_US.TRIG 3.56,42.29 3.56,45.47 7.62,49.53 12.95,49.53 13.84,48.64 13.84,42.67 16.76,39.75 32.51,39.75 33.66,40.89 49.4,40.89 50.93,39.37 FRDM1.PTC16
USR_LED  (via drill 0.7 pad 1.02)
  46 0.406: v47.5,57.91 45.85,57.91 41.91,53.98 41.91,49.4 39.88,47.37 39.88,44.07 38.99,43.18 37.34,43.18 36.83,42.67 v36.83,38.35 | v36.45,26.54 36.45,7.49 39.37,4.57 LED_U1.K
  Bottom 0.406: v47.5,57.91 50.29,60.96 52.07,60.96 FRDM1.PTC0 | v36.83,38.35 35.31,36.83 35.31,29.84 36.45,28.7 v36.45,26.54
V_IN  (via drill 0.7, 0.9 pad 1.42)  (1 unrouted)
  46 0.406: R4.2 15.88,12.45 v15.24,13.08 | BUTTON_ON.2 9.4,1.78 J_BATT_1.+
  46 0.61: 31.37,41.21 C13.2
  46 0.813: v28.45,18.54 28.45,32.38 28.57,32.38 31.11,34.92 31.43,35.24 | 37.62,45.88 35.31,43.56 35.31,39.12 | 35.31,39.12 35.31,37.47 36.45,36.32 38.38,36.32 | 28.19,18.8 v28.45,18.54 | FET_P.2 26.24,20.75 v28.45,18.54 | 31.43,35.24 35.31,39.12 | 31.37,41.21 31.37,38.41 C15.2 31.43,35.24
  46 1.016: C18.+ 37.62,45.88 | 38.38,36.32 C19.+
  Bottom 0.406: v15.24,13.08 15.24,12.7 13.97,11.43
  Bottom 0.813: 10.54,2.92 10.54,8 13.97,11.43 21.34,11.43 v28.45,18.54
VDD  (via drill 0.9 pad 1.42)
  46 0.406: R7.2 28.06,10.28 30.48,12.7 30.48,14.63 D_1.2
  46 0.61: v8.89,18.03 8.89,14.92 R5.2 | D_2.1 13.02,27.62 13.97,26.67 | 23.11,18.03 23.75,17.4 27.71,17.4 D_1.2
  46 0.813: FET_P.1 v22.86,18.03 23.11,18.03 | v8.89,18.03 8.89,21.59 13.97,26.67 15.49,28.19 15.49,33.53 16.89,34.92 16.89,45.47 J_REG_5V.VIN
  Bottom 0.813: v22.86,18.03 v8.89,18.03 | J_REG_5V.VIN 17.14,44.32 18.54,42.93 30.48,42.93 31.75,44.2 J_REG_9V.VIN

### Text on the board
tNames: Version / 09.09.13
